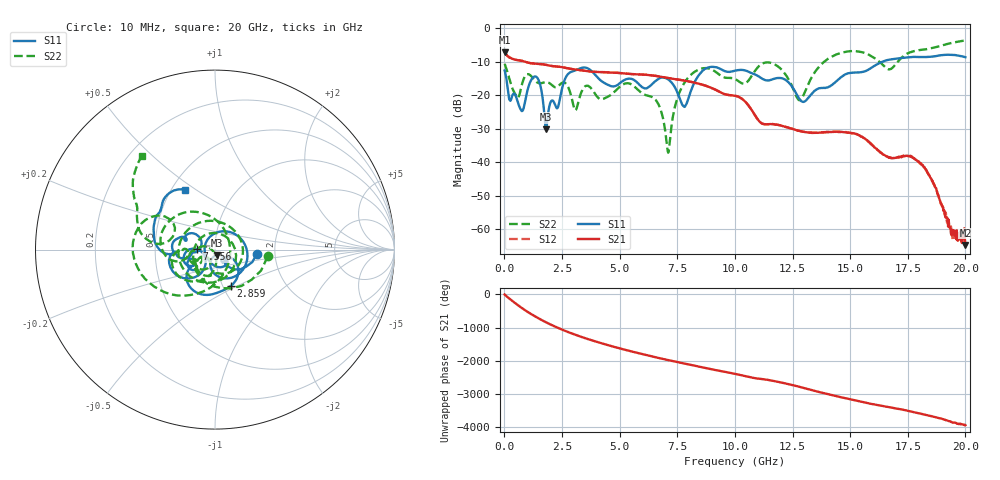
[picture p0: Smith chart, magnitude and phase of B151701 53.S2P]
!  2-Port S-parameters saved by WinCal
! VAR MeasName=S-Parameters (CALIBRATED_DATA) read from VNA (N5244A)
! VAR MeasDate=2015-12-24 19:16:09
! VAR NAME=B151701 53
! VAR FILENAME=B151701 53.S2P
! VAR DATE=2015-12-24 19:16:09
! VAR PHYS_PORTS=1,3
# Hz S DB R 50
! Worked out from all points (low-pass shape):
!   801 points, 10 MHz to 20 GHz, reference 50 ohm
!   highest |S21| = -7.11 dB at 10 MHz (marker M1); lowest = -64.7 dB at 20 GHz (marker M2)
!   |S21| within 3 dB of the highest: start of sweep to 965.4 MHz
!   lowest |S11| = -30.1 dB at 1.809 GHz (marker M3), VSWR 1.06, Z = 50.9 - j3 ohm
!   |S11| at or under -10 dB: start of sweep to 16.38 GHz
!   |S22| runs from -37.2 to -3.6 dB; largest |S21 - S12| = 0.0012
!   S11 on the Smith chart (normalised r, x): 10 MHz: 1.61, -0.08; 2.859 GHz: 1.09, -0.47; 7.556 GHz: 0.82, +0.00; 20 GHz: 0.59, +0.45
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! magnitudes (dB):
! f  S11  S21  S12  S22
! 10 MHz  -12.6  -7.1  -7.1  -10.6
! 734.6 MHz  -24.6  -9.7  -9.6  -17.5
! 1.409 GHz  -14.6  -10.6  -10.6  -16.1
! 1.809 GHz  -30.1  -10.9  -10.9  -16.1
! 2.859 GHz  -13.1  -12.1  -12.1  -19.3
! 3.083 GHz  -12.5  -12.3  -12.2  -24.5
! 3.358 GHz  -11.8  -12.5  -12.5  -18.8
! 5.382 GHz  -15.0  -13.6  -13.6  -16.4
! 6.682 GHz  -15.1  -14.3  -14.3  -22.6
! 7.106 GHz  -15.3  -14.8  -14.8  -37.2
! 7.556 GHz  -19.9  -15.3  -15.3  -19.8
! 7.856 GHz  -23.1  -15.7  -15.7  -15.7
! 8.531 GHz  -13.1  -16.7  -16.7  -12.0
! 10.01 GHz  -12.6  -20.1  -20.1  -15.1
! 11.58 GHz  -15.3  -28.6  -28.6  -10.3
! 12.8 GHz  -21.1  -30.6  -30.7  -21.5
! 13.35 GHz  -19.4  -31.2  -31.2  -14.3
! 14.98 GHz  -13.3  -31.2  -31.2  -6.8
! 16.68 GHz  -9.4  -38.5  -38.5  -12.3
! 18.15 GHz  -8.6  -40.9  -41.0  -6.3
! 19.35 GHz  -7.9  -59.7  -59.3  -4.4
! 20 GHz  -8.6  -64.7  -65.1  -3.6
